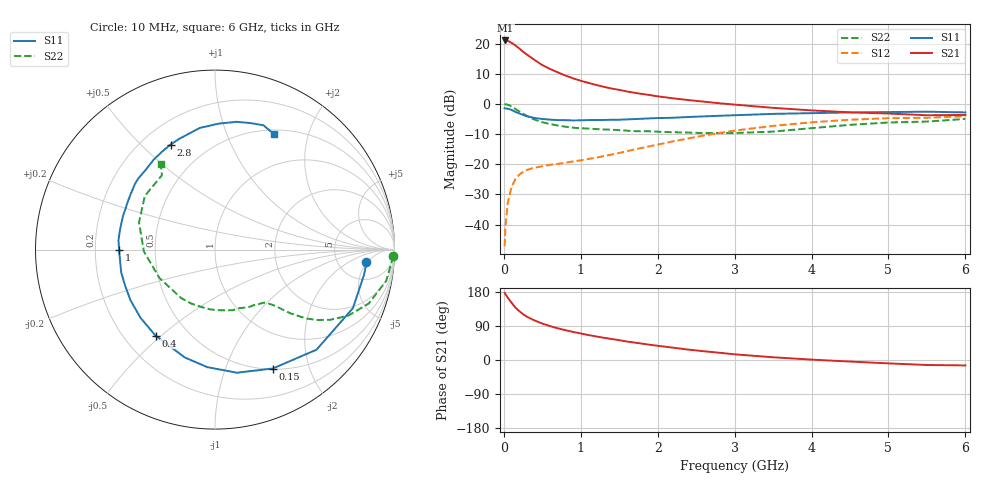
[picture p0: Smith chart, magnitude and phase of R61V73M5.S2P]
! SIEMENS Small Signal Semiconductors
! BFR193
! Si NPN RF Bipolar Junction Transistor in SOT23
! VCE = 1.75 V  IC = 3.5 mA
! Common Emitter S-Parameters:  May  1996
# GHz  S  MA  R  50
!  f  S11  S21  S12  S22
! GHz  MAG  ANG  MAG  ANG  MAG  ANG  MAG  ANG
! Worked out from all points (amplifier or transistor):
!   36 points, 10 MHz to 6 GHz, reference 50 ohm
!   highest |S21| = 21.0 dB at 20 MHz (marker M1)
!   |S21| within 3 dB of that: start of sweep to 216 MHz
!   unconditionally stable (mu >= 1): 982.8 MHz to 2.044 GHz
!   at 250 MHz: K = 0.34, MSG = 19.9 dB, |S12| = -22.5 dB
!   at 1.4 GHz: K = 1.09, MAG = 9.1 dB, |S12| = -16.8 dB
!   at 6 GHz: K = 0.98, MSG = 0.2 dB, |S12| = -4.1 dB
!   S11 on the Smith chart (normalised r, x): 10 MHz: 10, -5; 150 MHz: 0.51, -1.47; 400 MHz: 0.33, -0.48; 1 GHz: 0.30, -0.00; 2.8 GHz: 0.31, +0.62; 6 GHz: 0.55, +1.48
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0.01  0.8467 -4.7  11.12 177.3  0.0044 84.6  0.9947 -2.1
0.02  0.8427 -9.3  11.24 173.8  0.0089 84.4  0.9861 -4.1
0.05  0.8348 -23.0  11.12 164.8  0.0227 77.5  0.9695 -10.4
0.1  0.7943 -44.6  10.25 151.3  0.042 68.0  0.9078 -19.3
0.15  0.7365 -64.1  9.326 138.4  0.0567 59.1  0.8285 -26.4
0.2  0.6967 -79.9  8.282 128.9  0.067 52.9  0.751 -31.4
0.25  0.6564 -93.7  7.307 120.9  0.0749 48.4  0.687 -34.8
0.3  0.6241 -105.6  6.558 114.1  0.0806 45.3  0.6335 -37.2
0.4  0.5828 -124.6  5.337 104.3  0.0878 41.8  0.5495 -40.2
0.5  0.5628 -137.5  4.396 96.2  0.0927 40.5  0.4969 -41.8
0.6  0.5489 -149.2  3.789 89.6  0.0977 40.8  0.4645 -42.8
0.7  0.5391 -158.9  3.336 83.7  0.1016 41.8  0.4388 -44.2
0.8  0.5379 -166.4  2.95 78.7  0.1061 43.3  0.4189 -45.6
1  0.5345 -179.7  2.414 69.9  0.1163 46.9  0.3961 -48.9
1.1  0.54 174.5  2.225 65.9  0.1224 48.7  0.3897 -51.2
1.6  0.5534 151.7  1.605 48.8  0.1643 56.1  0.3603 -64.2
2.2  0.5894 130.6  1.237 32.5  0.2397 57.1  0.3394 -85.2
2.8  0.6354 112.9  1.025 19.2  0.3295 51.7  0.3284 -113.9
3.5  0.6833 97.1  0.86 7.2  0.4321 40.2  0.3477 -153.0
4.5  0.7218 80.5  0.726 -4.1  0.5469 22.2  0.4498 160.3
5.5  0.7434 68.7  0.649 -13.2  0.5889 4.5  0.5092 125.5
6  0.7227 63.1  0.656 -14.3  0.6245 -0.5  0.5641 122.4
